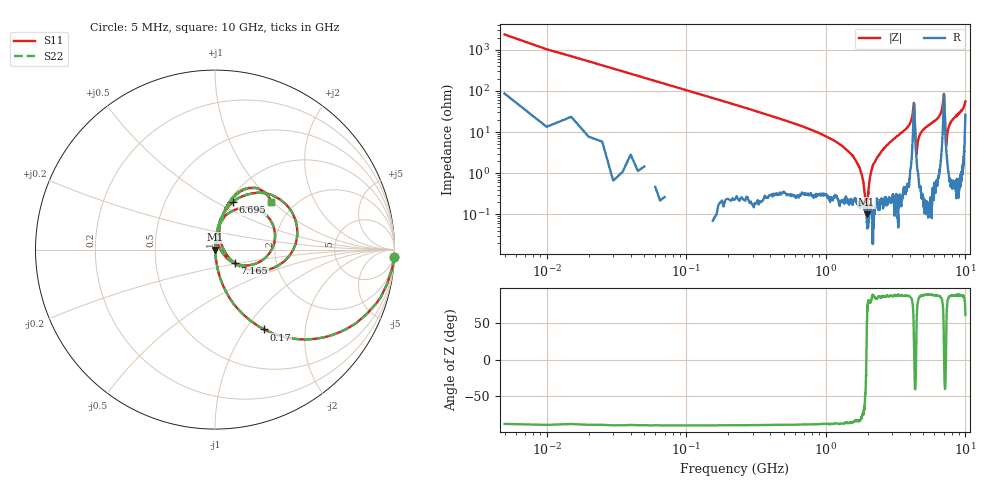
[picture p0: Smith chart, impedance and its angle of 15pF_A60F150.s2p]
! Amotech Co.,Ltd.
! http://www.amotech.co.kr/
! Part Number: A60F150
! These Parameters are Measured in Series Mode Connection
! Operation Temp=25[degC], DC Bias Voltage=0[V]
! Freq. Start=5[MHz] Stop=10[GHz], 2000[Steps]
! Date: Monday, July 20, 2020, 04:10:51
# GHZ S RI R 50.000000
!Freq.(Hz) S11(Real) S11(Imag) S21(Real) S21(Imag) S12(Real) S12(Imag) S22(Real) S22(Imag)
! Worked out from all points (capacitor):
!   2000 points, 5 MHz to 10 GHz, reference 50 ohm
!   read as one part in series: C = 15.2 pF near 55 MHz
!   lowest |Z| = 99.4 mohm at 1.96 GHz (marker M1)
!   series resonance near 1.951 GHz, so ESL is about 440 pH
!   S11 on the Smith chart (normalised r, x): 5 MHz: 3, -47; 170 MHz: 1.00, -1.23; 6.695 GHz: 1.05, +0.60; 7.165 GHz: 1.23, -0.19; 10 GHz: 1.53, +0.98
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0.005  0.9967 -0.0419  0.0033 0.0419  0.0033 0.0419  0.9967 -0.0419
0.075  0.6612 -0.4733  0.3388 0.4733  0.3388 0.4733  0.6612 -0.4733
0.17  0.2739 -0.4446  0.7261 0.4446  0.7261 0.4446  0.2739 -0.4446
0.475  0.0447 -0.1992  0.9553 0.1992  0.9553 0.1992  0.0447 -0.1992
1.675  0.00243 -0.0176  0.9976 0.0176  0.9976 0.0176  0.00243 -0.0176
1.82  0.00216 -0.00816  0.9978 0.00816  0.9978 0.00816  0.00216 -0.00816
1.96  0.000941 0.000315  0.9991 -0.000315  0.9991 -0.000315  0.000941 0.000315
2.09  0.00167 0.00918  0.9983 -0.00918  0.9983 -0.00918  0.00167 0.00918
2.215  0.00112 0.0172  0.9989 -0.0172  0.9989 -0.0172  0.00112 0.0172
3.34  0.00963 0.084  0.9904 -0.084  0.9904 -0.084  0.00963 0.084
4.255  0.2767 0.2006  0.7233 -0.2006  0.7233 -0.2006  0.2767 0.2006
4.46  0.0222 0.0167  0.9778 -0.0167  0.9778 -0.0167  0.0222 0.0167
4.65  0.0114 0.0742  0.9886 -0.0742  0.9886 -0.0742  0.0114 0.0742
5.005  0.0153 0.1138  0.9847 -0.1138  0.9847 -0.1138  0.0153 0.1138
6.67  0.0947 0.2586  0.9053 -0.2586  0.9053 -0.2586  0.0947 0.2586
6.695  0.1009 0.2648  0.8991 -0.2648  0.8991 -0.2648  0.1009 0.2648
7.01  0.4573 0.1214  0.5427 -0.1214  0.5427 -0.1214  0.4573 0.1214
7.165  0.1117 -0.0763  0.8883 0.0763  0.8883 0.0763  0.1117 -0.0763
7.285  0.0379 0.0241  0.9621 -0.0241  0.9621 -0.0241  0.0379 0.0241
7.625  0.0269 0.1329  0.9731 -0.1329  0.9731 -0.1329  0.0269 0.1329
8.335  0.0533 0.2117  0.9467 -0.2117  0.9467 -0.2117  0.0533 0.2117
10  0.3133 0.2672  0.6867 -0.2672  0.6867 -0.2672  0.3133 0.2672
